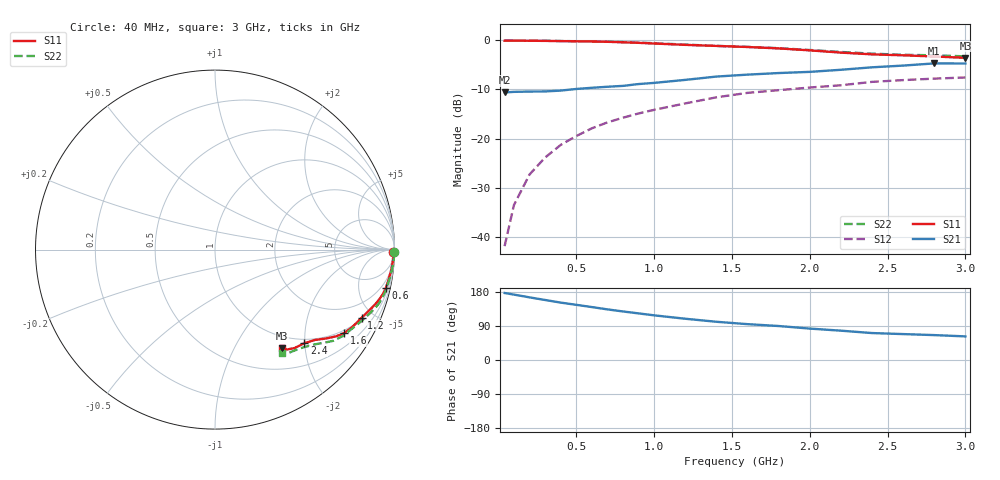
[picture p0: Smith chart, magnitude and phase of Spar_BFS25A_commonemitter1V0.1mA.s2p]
! Filename:  BFS25AA.S2P  Version:  4.0
! NXP part #: BFS25A  Date: Jun 1994
! Bias condition: Vce=1V, Ic=0.1mA
#  MHz  S  MA  R  50
! Freq  S11  S21  S12  S22  !GUM [dB]
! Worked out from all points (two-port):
!   21 points, 40 MHz to 3 GHz, reference 50 ohm
!   highest |S21| = -4.69 dB at 2.8 GHz (marker M1); lowest = -10.6 dB at 40 MHz (marker M2)
!   |S21| within 3 dB of the highest: 1.307 GHz to end of sweep
!   lowest |S11| = -3.6 dB at 3 GHz (marker M3), VSWR 4.95, Z = 40 - j78.8 ohm
!   |S11| at or under -10 dB: nowhere
!   |S22| runs from -3.2 to 0.0 dB; largest |S21 - S12| = 0.3
!   S11 on the Smith chart (normalised r, x): 40 MHz: open; 600 MHz: 1.01, -8.80; 1.2 GHz: 1.06, -4.28; 1.6 GHz: 0.90, -3.15; 2.4 GHz: 0.92, -1.99; 3 GHz: 0.80, -1.58
40  0.994 -0.8  0.295 176.8  0.008 87.3  0.999 -0.9
100  0.994 -2.0  0.299 172.6  0.021 86.4  0.998 -2.3
200  0.992 -4.1  0.301 165.3  0.043 84.1  0.995 -4.6
300  0.989 -6.3  0.302 158.4  0.064 81.6  0.991 -6.9
400  0.984 -8.5  0.308 151.5  0.086 79.9  0.986 -9.3
500  0.98 -10.7  0.32 145.6  0.106 78.0  0.981 -11.7
600  0.975 -12.8  0.329 139.7  0.127 76.2  0.977 -13.9
700  0.968 -14.8  0.337 133.6  0.146 74.4  0.97 -16.1
800  0.957 -16.7  0.344 128.1  0.163 72.4  0.962 -18.1
900  0.945 -18.6  0.359 123.0  0.18 70.1  0.95 -20.0
1000  0.93 -20.6  0.369 117.9  0.196 67.8  0.936 -22.0
1200  0.901 -24.9  0.396 108.9  0.228 63.1  0.907 -26.2
1400  0.879 -29.3  0.428 100.9  0.263 59.2  0.879 -30.4
1600  0.857 -32.9  0.448 94.6  0.292 55.5  0.859 -34.1
1800  0.829 -35.7  0.465 89.7  0.311 53.2  0.834 -37.5
2000  0.792 -38.7  0.478 82.9  0.331 49.7  0.799 -40.5
2200  0.751 -42.1  0.502 77.4  0.349 46.5  0.763 -43.9
2400  0.721 -46.3  0.532 71.1  0.378 42.7  0.733 -48.1
2600  0.705 -51.1  0.554 68.4  0.394 39.8  0.714 -52.2
2800  0.686 -54.3  0.583 65.7  0.408 38.9  0.705 -55.3
3000  0.664 -56.0  0.582 62.3  0.419 36.8  0.688 -57.2
